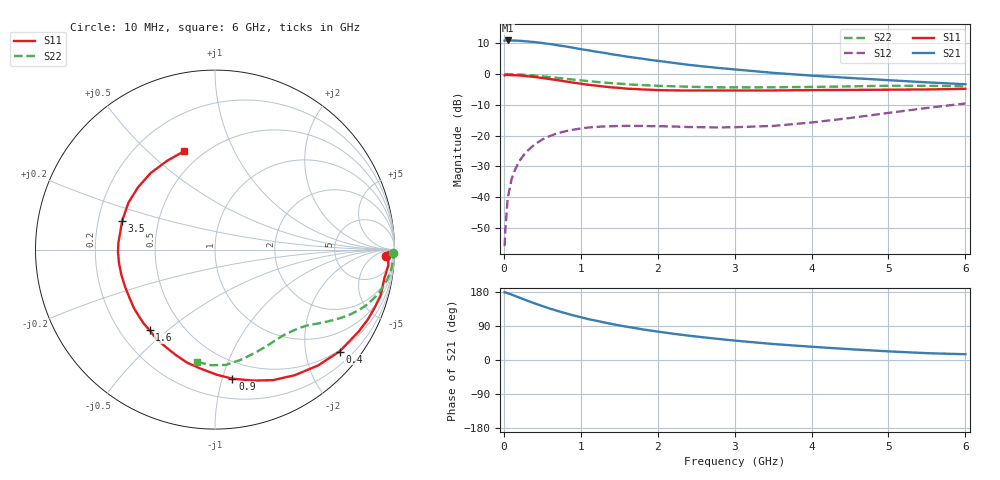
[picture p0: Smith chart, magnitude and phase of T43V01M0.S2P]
! Infineon Technologies  Discrete & RF Semiconductors
! BFR182T
! Si NPN RF Bipolar Junction Transistor in SC75
! VCE = 3 V  IC = 1 mA
! Common Emitter S-Parameters:  October  1999
# GHz  S  MA  R  50
!  f  S11  S21  S12  S22
! GHz  MAG  ANG  MAG  ANG  MAG  ANG  MAG  ANG
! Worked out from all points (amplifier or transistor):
!   36 points, 10 MHz to 6 GHz, reference 50 ohm
!   highest |S21| = 10.9 dB at 50 MHz (marker M1)
!   |S21| within 3 dB of that: start of sweep to 1.046 GHz
!   unconditionally stable (mu >= 1): 2.382 GHz to 4.561 GHz
!   at 250 MHz: K = 0.10, MSG = 18.7 dB, |S12| = -26.6 dB
!   at 1.4 GHz: K = 0.58, MSG = 11.7 dB, |S12| = -17.0 dB
!   at 6 GHz: K = 0.84, MSG = 3.1 dB, |S12| = -9.6 dB
!   S11 on the Smith chart (normalised r, x): 10 MHz: 27, -22; 400 MHz: 0.47, -2.73; 900 MHz: 0.36, -1.08; 1.6 GHz: 0.32, -0.43; 3.5 GHz: 0.30, +0.14; 6 GHz: 0.40, +0.65
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0.01  0.956 -2.1  3.489 178.7  0.0016 87.6  0.9916 -1.1
0.02  0.9654 -0.8  3.495 178.8  0.003 99.4  0.9999 -0.8
0.05  0.9694 -5.2  3.513 176.2  0.0096 88.0  0.9967 -2.0
0.1  0.9569 -9.7  3.495 172.7  0.0195 86.6  0.9934 -3.9
0.15  0.9577 -15.3  3.489 168.6  0.0288 81.9  0.9894 -5.8
0.25  0.9361 -24.6  3.43 160.9  0.0468 75.2  0.9757 -9.5
0.4  0.8965 -39.3  3.306 149.4  0.0719 67.1  0.945 -14.8
0.5  0.864 -48.3  3.192 142.4  0.0865 62.2  0.9201 -17.7
0.6  0.8294 -57.5  3.071 135.6  0.0987 57.8  0.8936 -20.6
0.7  0.7957 -66.1  2.936 129.4  0.1096 53.6  0.8656 -23.1
0.8  0.759 -74.0  2.814 123.6  0.1177 49.6  0.8387 -25.4
0.9  0.7256 -82.3  2.676 118.0  0.1247 46.5  0.8125 -27.4
1.1  0.6681 -96.9  2.43 107.9  0.1356 40.5  0.7668 -30.8
1.4  0.608 -116.8  2.099 95.2  0.1419 34.3  0.7128 -35.1
1.6  0.5784 -129.1  1.919 87.7  0.1441 31.8  0.6839 -37.5
1.8  0.5618 -139.9  1.777 80.9  0.1435 30.3  0.6604 -40.0
2.2  0.5424 -157.4  1.522 69.4  0.1407 29.7  0.6333 -44.6
2.8  0.5408 -178.3  1.253 55.4  0.1359 34.4  0.6091 -52.7
3.5  0.5413 162.9  1.046 42.2  0.1437 45.6  0.6103 -62.1
4.5  0.5519 141.0  0.864 28.5  0.1933 58.1  0.6305 -76.8
5.5  0.5621 118.5  0.733 18.0  0.2812 60.1  0.6445 -91.8
6  0.5742 107.7  0.683 15.2  0.3328 57.4  0.6335 -98.9
